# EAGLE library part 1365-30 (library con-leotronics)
DUAL ROW STRAIGHT HEADER 1364 SERIES. 1.27mm x 1.27mm. Without Fixing Post. SMT Source: http://www.leotronics.co.uk/Conexcon/Data%20Sheets/sec.%20A/1364ing.pdf
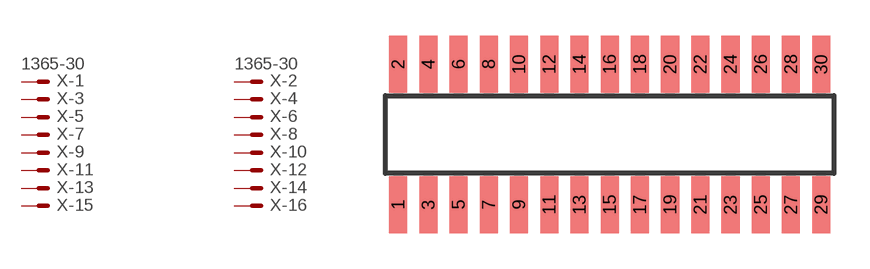
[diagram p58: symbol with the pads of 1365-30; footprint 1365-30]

Designator prefix X; gates -1=MVAL -2=MVAL -3=M -4=M -5=M -6=M -7=M -8=M -9=M -10=M -11=M -12=M -13=M -14=M -15=M -16=M -17=M -18=M -19=M -20=M -21=M -22=M -23=M -24=M -25=M -26=M -27=M -28=M -29=M -30=M

## 1365-30 (OC_FARNELL: unknown; OC_NEWARK: unknown)  [1365-30]
1  -1:S  pas
2  -2:S  pas
3  -3:S  pas
4  -4:S  pas
5  -5:S  pas
6  -6:S  pas
7  -7:S  pas
8  -8:S  pas
9  -9:S  pas
10  -10:S  pas
11  -11:S  pas
12  -12:S  pas
13  -13:S  pas
14  -14:S  pas
15  -15:S  pas
16  -16:S  pas
17  -17:S  pas
18  -18:S  pas
19  -19:S  pas
20  -20:S  pas
21  -21:S  pas
22  -22:S  pas
23  -23:S  pas
24  -24:S  pas
25  -25:S  pas
26  -26:S  pas
27  -27:S  pas
28  -28:S  pas
29  -29:S  pas
30  -30:S  pas

## Footprint 1365-30 (pad centres in mm)
DUAL ROW STRAIGHT HEADER 1364 SERIES. 1.27mm x 1.27mm. Without Fixing Post. SMT Source: http://www.leotronics.co.uk/Conexcon/Data%20Sheets/sec.%20A/1364ing.pdf
smd 0.76 x 2.4: 1 -8.89,-2.95; 2 -8.89,2.95; 3 -7.62,-2.95; 4 -7.62,2.95; 5 -6.35,-2.95; 6 -6.35,2.95; 7 -5.08,-2.95; 8 -5.08,2.95; 9 -3.81,-2.95; 10 -3.81,2.95; 11 -2.54,-2.95; 12 -2.54,2.95; 13 -1.27,-2.95; 14 -1.27,2.95; 15 0,-2.95; 16 0,2.95; 17 1.27,-2.95; 18 1.27,2.95; 19 2.54,-2.95; 20 2.54,2.95; 21 3.81,-2.95; 22 3.81,2.95; 23 5.08,-2.95; 24 5.08,2.95; 25 6.35,-2.95; 26 6.35,2.95; 27 7.62,-2.95; 28 7.62,2.95; 29 8.89,-2.95; 30 8.89,2.95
